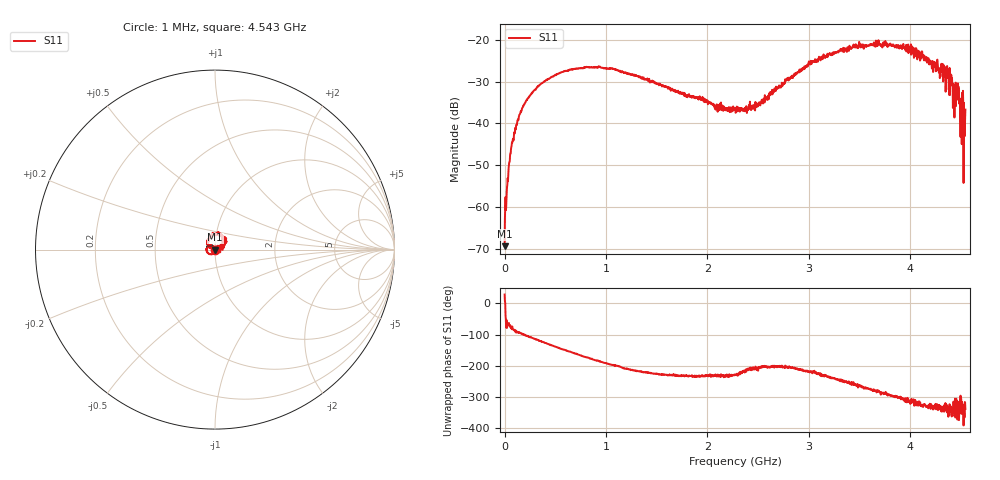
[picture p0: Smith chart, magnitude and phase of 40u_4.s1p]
# HZ S RI R 50
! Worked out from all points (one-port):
!   1515 points, 1 MHz to 4.543 GHz, reference 50 ohm
!   lowest |S11| = -69.4 dB at 1 MHz (marker M1), VSWR 1.00, Z = 50 + j0.0162 ohm
!   |S11| at or under -10 dB: start of sweep to end of sweep
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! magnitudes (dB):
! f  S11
! 1 MHz  -69.4
! 28 MHz  -54.6
! 61 MHz  -47.2
! 115 MHz  -40.5
! 163 MHz  -37.2
! 340 MHz  -30.9
! 571 MHz  -27.7
! 922 MHz  -26.6
! 1.138 GHz  -27.4
! 1.705 GHz  -32.5
! 1.972 GHz  -34.4
! 2.098 GHz  -36.7
! 2.272 GHz  -36.8
! 2.506 GHz  -35.4
! 2.842 GHz  -29.1
! 3.016 GHz  -25.3
! 3.409 GHz  -21.9
! 3.682 GHz  -20.2
! 3.976 GHz  -21.9
! 4.381 GHz  -28.2
! 4.429 GHz  -31.0
! 4.468 GHz  -30.4
! 4.486 GHz  -34.0
! 4.501 GHz  -42.7
! 4.504 GHz  -38.5
! 4.516 GHz  -35.5
! 4.531 GHz  -42.7
! 4.543 GHz  -36.7
